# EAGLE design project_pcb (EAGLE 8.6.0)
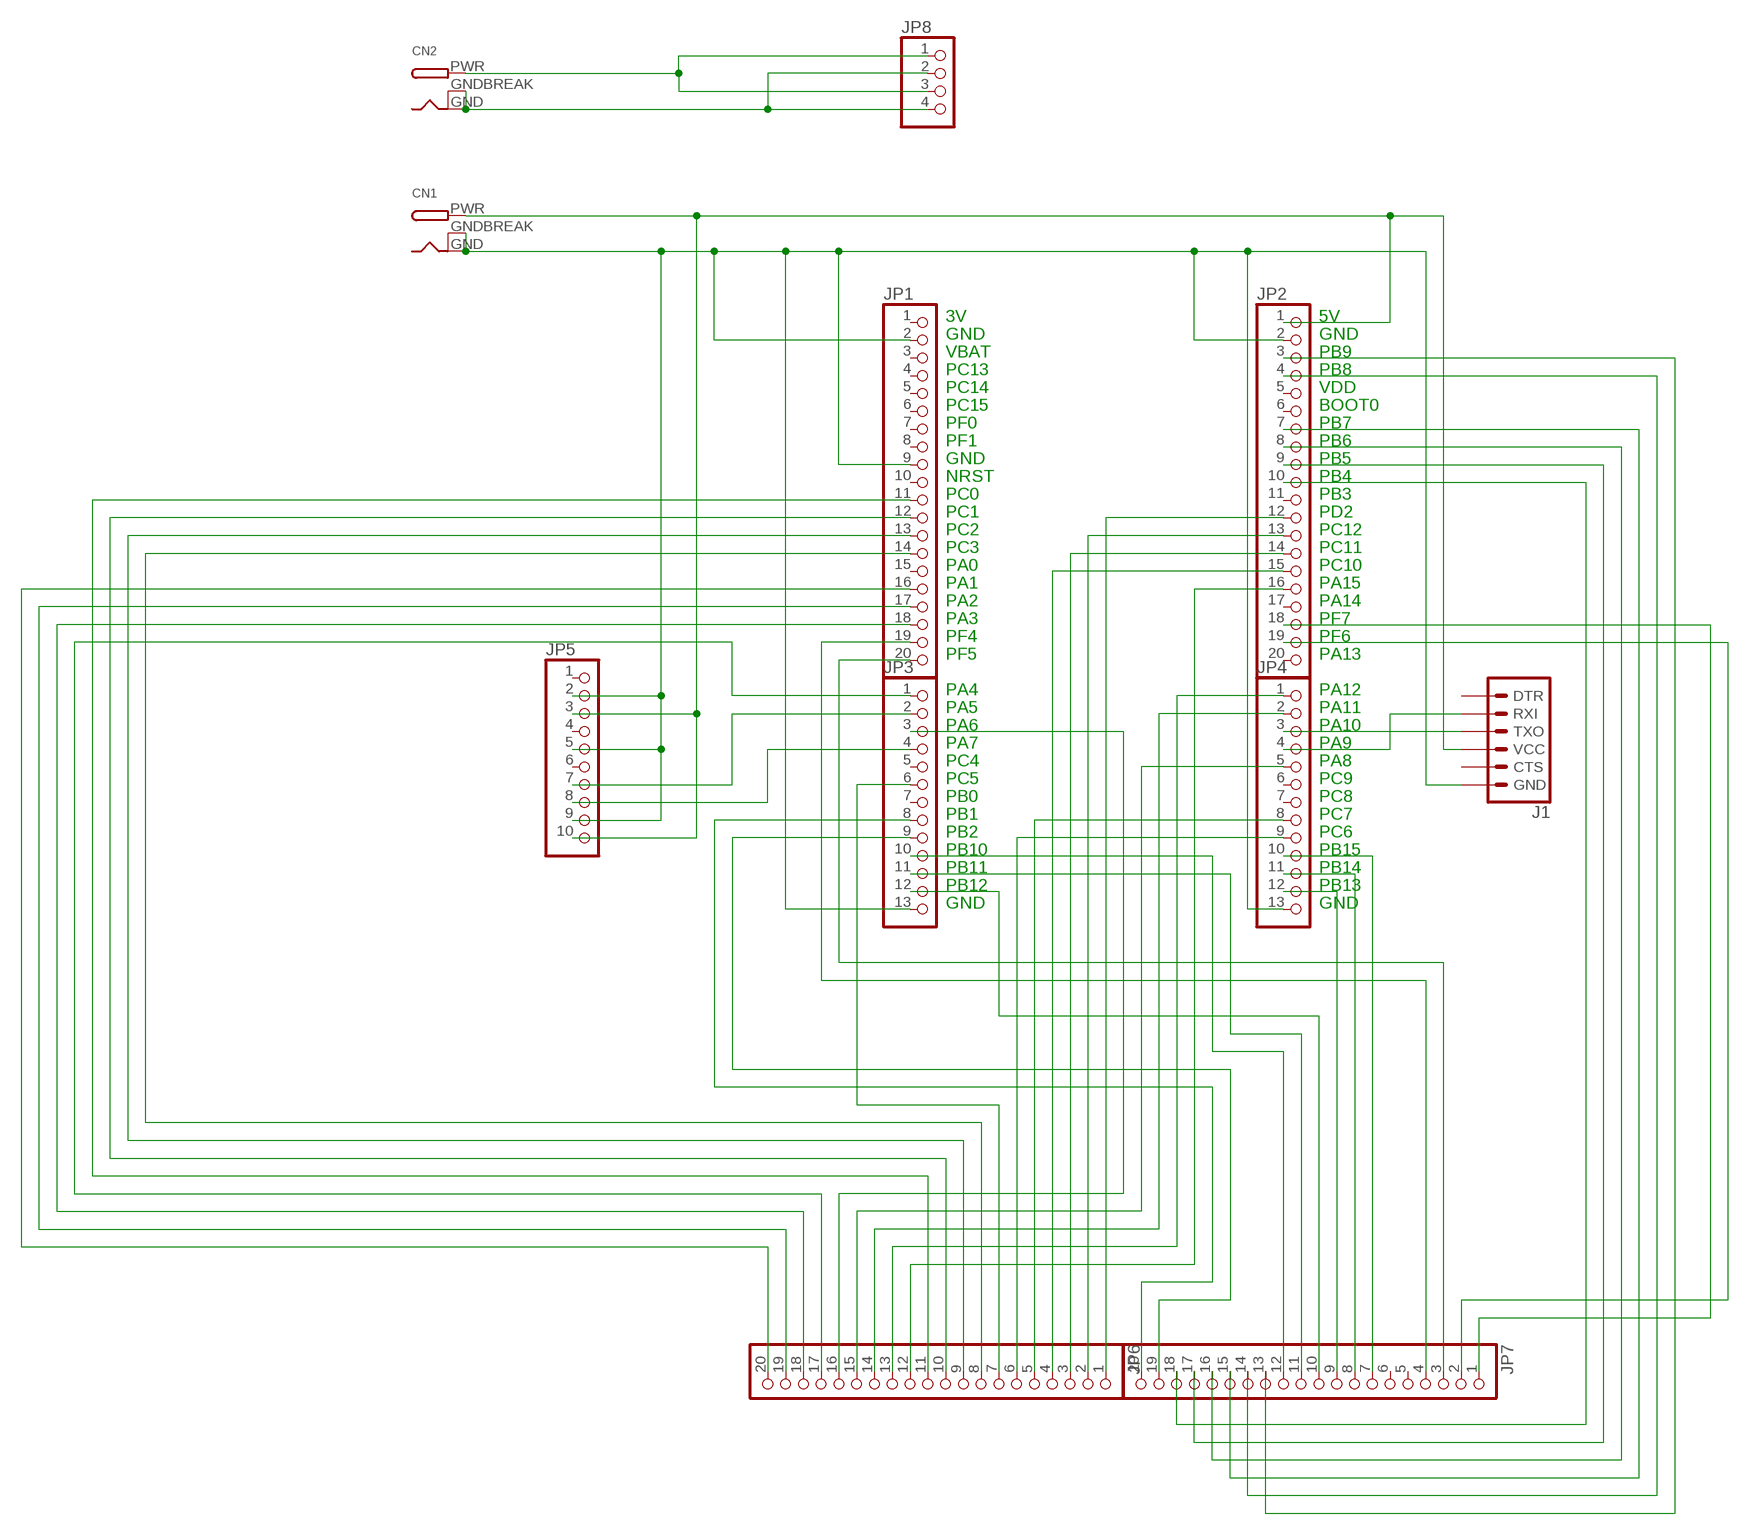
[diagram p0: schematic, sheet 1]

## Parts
CN1  DCBARRELPTH  [DCJACK_2MM_PTH]
CN2  DCBARRELPTH  [DCJACK_2MM_PTH]
J1  6_PIN_SERIAL_TARGET  [1X06]
JP1  PINHD-1X20  [1X20]
JP2  PINHD-1X20  [1X20]
JP3  PINHD-1X13  [1X13]
JP4  PINHD-1X13  [1X13]
JP5  PINHD-1X10  [1X10]
JP6  PINHD-1X20  [1X20]
JP7  PINHD-1X20  [1X20]
JP8  PINHD-1X4  [1X04]

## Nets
N$1: J1.3(TXO) JP4.3
N$2: J1.2(RXI) JP4.4
N$3: CN1.PWR J1.4(VCC) JP2.1 JP5.3 JP5.10
N$4: CN1.GND CN1.GNDBREAK J1.6(GND) JP1.2 JP1.9 JP2.2 JP3.13 JP4.13 JP5.2 JP5.5 JP5.9
N$5: JP3.2 JP5.7
N$6: JP3.4 JP5.8
N$7: JP1.16 JP6.20
N$8: JP1.17 JP6.19
N$9: JP1.18 JP6.18
N$10: JP3.1 JP6.17
N$11: JP3.3 JP6.16
N$12: JP4.5 JP6.15
N$13: JP4.2 JP6.14
N$14: JP4.1 JP6.13
N$15: JP2.16 JP6.12
N$16: JP1.11 JP6.11
N$17: JP1.12 JP6.10
N$18: JP1.13 JP6.9
N$19: JP1.14 JP6.8
N$20: JP3.6 JP6.7
N$21: JP4.9 JP6.6
N$22: JP4.8 JP6.5
N$23: JP2.15 JP6.4
N$24: JP2.14 JP6.3
N$25: JP2.13 JP6.2
N$26: JP2.10 JP7.18
N$27: JP3.8 JP7.20
N$28: JP3.9 JP7.19
N$29: JP2.9 JP7.17
N$30: JP2.8 JP7.16
N$31: JP2.7 JP7.15
N$32: JP2.4 JP7.14
N$33: JP2.3 JP7.13
N$34: JP3.10 JP7.12
N$35: JP3.11 JP7.11
N$36: JP3.12 JP7.10
N$37: JP4.12 JP7.9
N$38: JP4.11 JP7.8
N$39: JP4.10 JP7.7
N$40: JP2.18 JP7.1
N$41: JP2.19 JP7.2
N$42: JP1.20 JP7.3
N$43: JP1.19 JP7.4
N$44: JP2.12 JP6.1
N$45: CN2.GND CN2.GNDBREAK JP8.2 JP8.4
N$46: CN2.PWR JP8.1 JP8.3
Unconnected: J1.1(DTR) J1.5(CTS) JP1.1 JP1.3 JP1.4 JP1.5 JP1.6 JP1.7 JP1.8 JP1.10 JP1.15 JP2.5 JP2.6 JP2.11 JP2.17 JP2.20 JP3.5 JP3.7 JP4.6 JP4.7 JP5.1 JP5.4 JP5.6 JP7.5 JP7.6

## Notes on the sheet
- 3V | 5V
- GND | GND
- VBAT | PB9
- PC13 | PB8
- PC14 | VDD
- PC15 | BOOT0
- PF0 | PB7
- PF1 | PB6
- GND | PB5
- NRST | PB4
- PC0 | PB3
- PC1 | PD2
- PC2 | PC12
- PC3 | PC11
- PA0 | PC10
- PA1 | PA15
- PA2 | PA14
- PA3 | PF7
- PF4 | PF6
- PF5 | PA13
- PA4 | PA12
- PA5 | PA11
- PA6 | PA10
- PA7 | PA9
- PC4 | PA8
- PC5 | PC9
- PB0 | PC8
- PB1 | PC7
- PB2 | PC6
- PB10 | PB15
- PB11 | PB14
- PB12 | PB13
- GND | GND

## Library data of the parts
CN1 CN2 = adafruit:DCBARREL: 2.0mm DC Barrel Jack DCJACK_2MM_PTH - Through Hole Jack (4UConnector: 05537)
J1 = SparkFun-Connectors:6_PIN_SERIAL_TARGET: 6-pin header connection for use with the "FTDI BASIC" pinout - TARGET SIDE. Also known as "Arduino Serial Program Header". It is used to mate with our FTDI Basic serial programmers using the Arduino IDE. Note, this device has "TARGET" in the name. It is intended to be used on a design that contains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
JP1 JP2 JP6 JP7 = pinhead:PINHD-1X20: PIN HEADER
JP3 JP4 = pinhead:PINHD-1X13: PIN HEADER
JP5 = pinhead:PINHD-1X10: PIN HEADER
JP8 = pinhead:PINHD-1X4: PIN HEADER

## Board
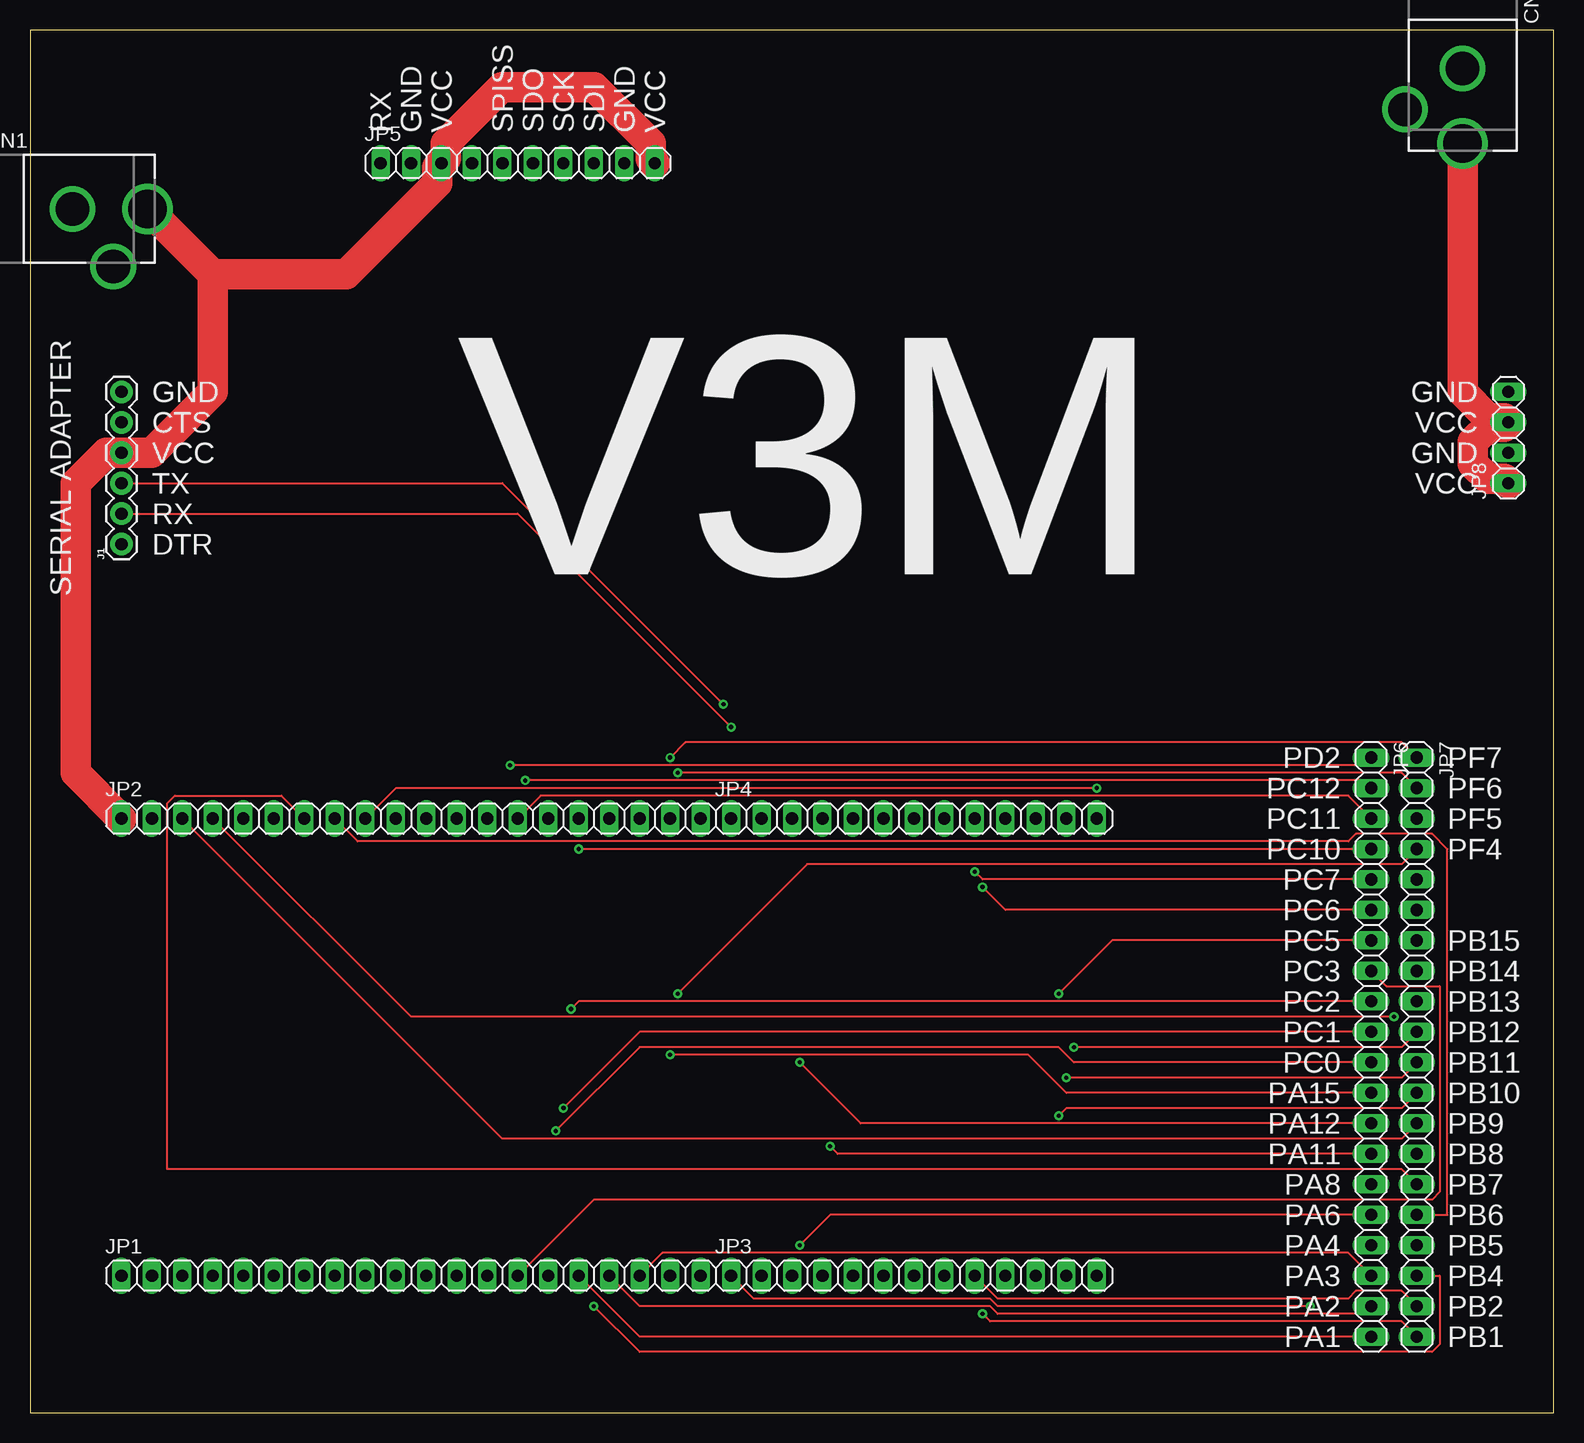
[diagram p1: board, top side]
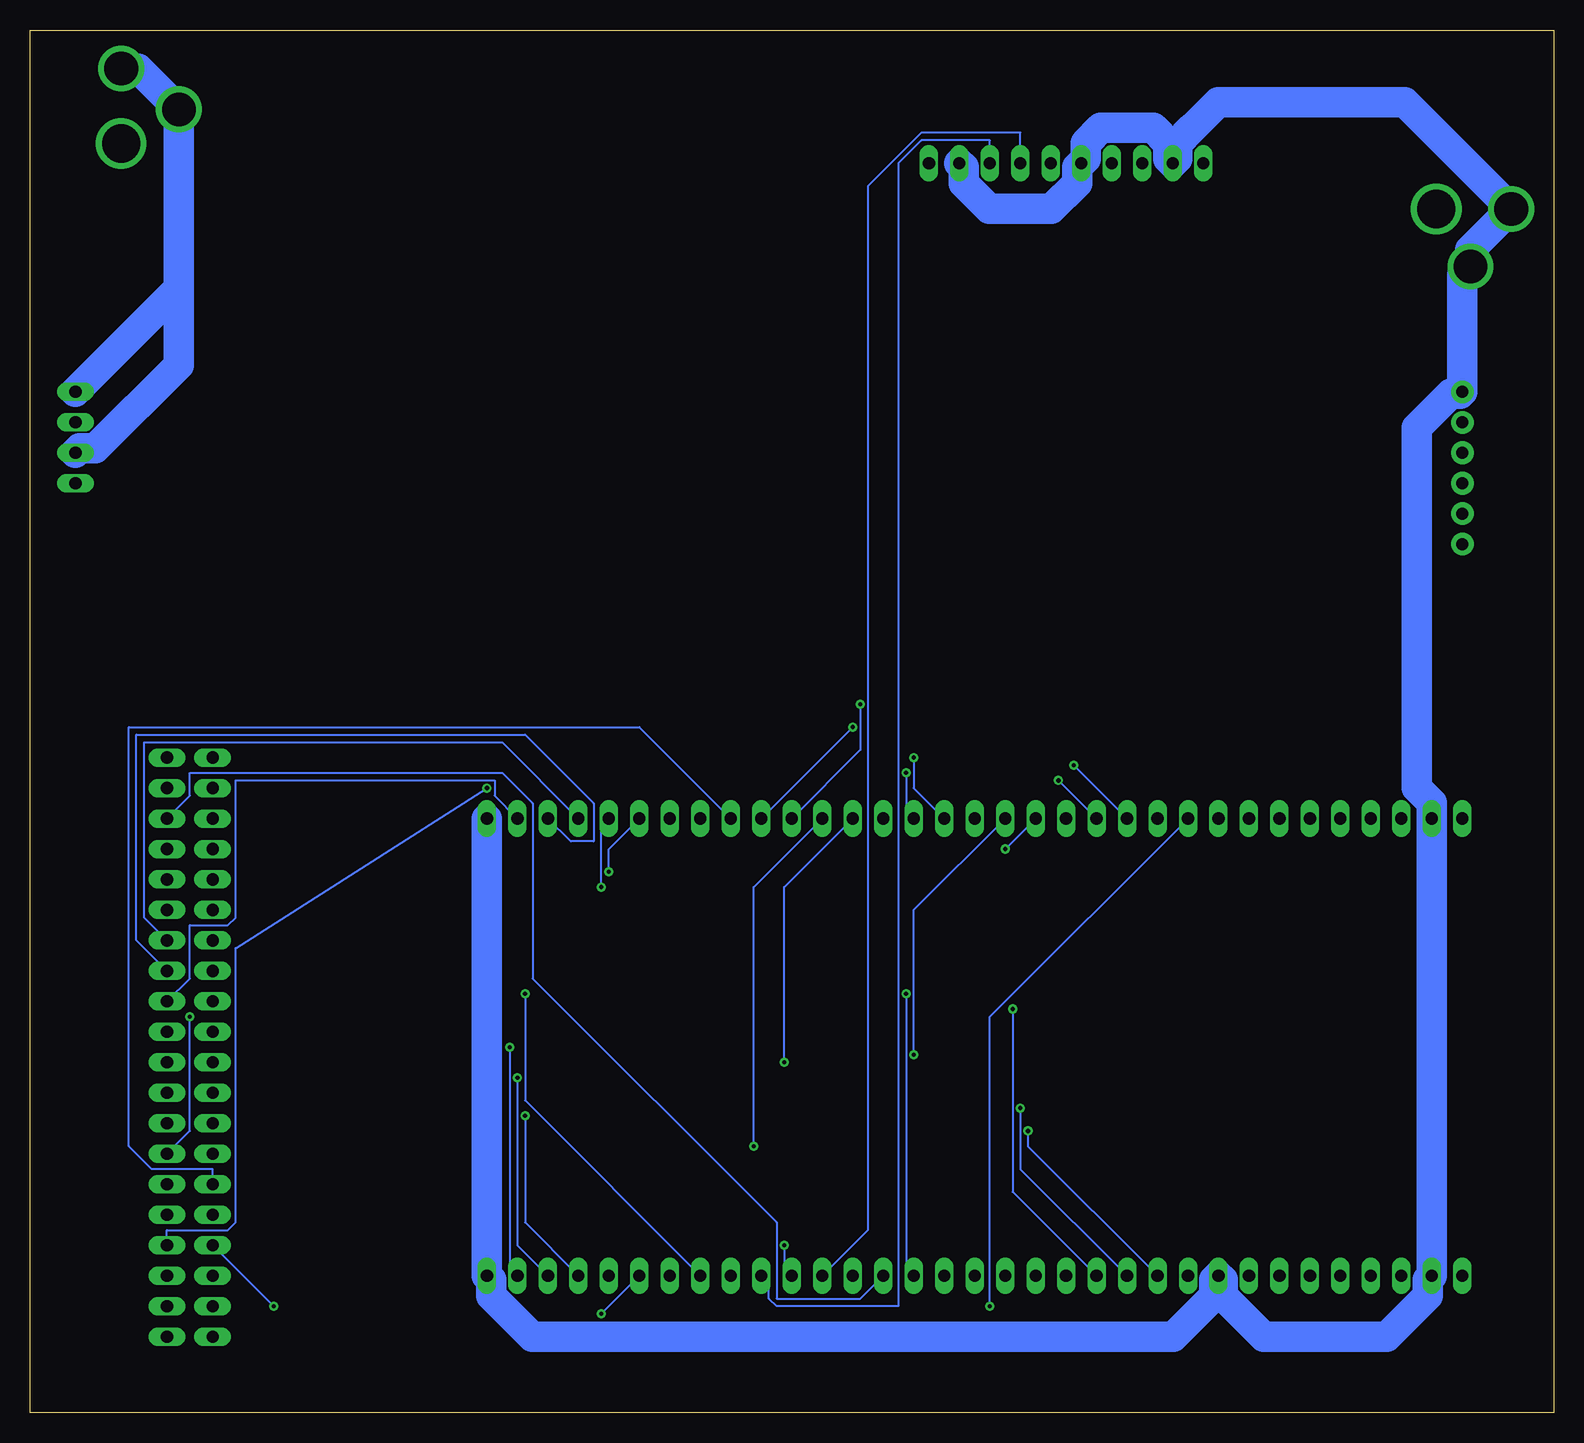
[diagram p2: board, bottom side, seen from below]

Size 126.98 x 115.24 mm. Coordinates in mm from the lower left corner, seen from the top.
Outline: 0,0 126.98,0 126.98,115.24 0,115.24 0,0
Copper layers (1*16): Top 0.035mm / dielectric 1.5mm / Bottom 0.035mm
Design rules "default": minimum track width 6mil, minimum drill 0.35mm, track to track 6mil, track to pad 6mil, pad to pad 6mil, via to via 6mil, smd to smd 6mil, copper to edge 40mil, drill to drill 6mil, minimum pad ring 10mil, minimum via ring 8mil, stop-mask expansion 4mil, vias tented up to drill 0mil, thermal gap 10mil

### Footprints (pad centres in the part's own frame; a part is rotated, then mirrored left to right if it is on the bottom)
DCJACK_2MM_PTH = drill 2.8: GND 0,7.35; GNDBREAK 4.8,10.75 | drill 3.2: PWR 0,13.6
1X06 = drill 1.016 pad 1.88: 1 0,0; 2 2.54,0; 3 5.08,0; 4 7.62,0; 5 10.16,0; 6 12.7,0
1X20 = drill 1.016 long: 1 -24.13,0; 2 -21.59,0; 3 -19.05,0; 4 -16.51,0; 5 -13.97,0; 6 -11.43,0; 7 -8.89,0; 8 -6.35,0; 9 -3.81,0; 10 -1.27,0; 11 1.27,0; 12 3.81,0; 13 6.35,0; 14 8.89,0; 15 11.43,0; 16 13.97,0; 17 16.51,0; 18 19.05,0; 19 21.59,0; 20 24.13,0
1X13 = drill 1.016 long: 1 -15.24,0; 2 -12.7,0; 3 -10.16,0; 4 -7.62,0; 5 -5.08,0; 6 -2.54,0; 7 0,0; 8 2.54,0; 9 5.08,0; 10 7.62,0; 11 10.16,0; 12 12.7,0; 13 15.24,0
1X10 = drill 1.016 long: 1 -11.43,0; 2 -8.89,0; 3 -6.35,0; 4 -3.81,0; 5 -1.27,0; 6 1.27,0; 7 3.81,0; 8 6.35,0; 9 8.89,0; 10 11.43,0
1X04 = drill 1.016 long: 1 -3.81,0; 2 -1.27,0; 3 1.27,0; 4 3.81,0

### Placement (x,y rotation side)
CN1  -3.81,100.33 270 top
CN2  119.38,119.38 180 top
J1  7.62,72.39 90 top
JP1  31.75,11.43 0 top
JP2  31.75,49.53 0 top
JP3  73.66,11.43 0 top
JP4  73.66,49.53 0 top
JP5  40.64,104.14 0 top
JP6  111.76,30.48 270 top
JP7  115.57,30.48 270 top
JP8  123.19,81.28 90 top

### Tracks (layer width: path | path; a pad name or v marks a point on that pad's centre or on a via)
N$1  (via drill 0.35)
  Top 0.152: v57.78,59.05 39.37,77.47 J1.3
  Bottom 0.152: JP4.3 57.78,55.24 v57.78,59.05
N$2  (via drill 0.35)
  Top 0.152: v58.42,57.15 40.64,74.93 J1.2
  Bottom 0.152: v58.42,57.15 JP4.4
N$3
  Top 2.54: CN1.PWR 15.24,94.88 | 15.24,94.88 15.24,85.09 10.16,80.01 J1.4 6.35,80.01 3.81,77.47 3.81,53.34 JP2.1 | 15.24,94.88 26.34,94.88 33.93,102.47 33.93,103.78 JP5.3 34.65,104.5 34.65,105.81 39.33,110.49 47.03,110.49 51.71,105.81 51.71,104.5 JP5.10
N$4
  Bottom 2.54: JP4.13 JP3.13 88.54,11.07 88.54,9.76 85.13,6.35 31.71,6.35 28.3,9.76 28.3,11.07 JP1.9 27.58,11.07 27.58,9.76 24.17,6.35 13.93,6.35 10.52,9.76 10.52,11.07 JP1.2 JP2.2 10.16,50.84 11.41,52.09 11.41,82.1 8.6,84.91 7.8,84.91 J1.6 7.62,94.85 CN1.GNDBREAK 6.94,96.93 CN1.GND 12.43,109.22 27.94,109.22 30.07,107.09 30.11,107.09 31.39,105.81 31.39,104.5 JP5.2 32.11,104.5 32.11,105.81 33.38,107.09 37.73,107.09 39.01,105.81 39.01,104.5 JP5.5 39.73,103.78 39.73,102.47 41.87,100.33 47.03,100.33 49.17,102.47 49.17,103.78 JP5.9
N$5
  Bottom 0.152: JP3.2 57.15,15.24 57.15,102.23 52.7,106.68 44.45,106.68 JP5.7
N$6
  Bottom 0.152: JP3.4 65.41,10.79 65.41,9.53 64.77,8.89 54.61,8.89 54.61,104.14 52.7,106.05 46.99,106.05 JP5.8
N$7
  Top 0.152: JP1.16 50.8,6.35 JP6.20
N$8
  Top 0.152: JP1.17 50.8,8.89 80.01,8.89 80.64,8.26 111.12,8.26 JP6.19
N$9
  Top 0.152: JP1.18 52.7,13.34 109.86,13.34 JP6.18
N$10  (via drill 0.35)
  Top 0.152: JP3.1 60.33,9.53 80.01,9.53 80.64,8.89 v106.68,8.89
  Bottom 0.152: JP6.17 v106.68,8.89
N$11  (via drill 0.35)
  Top 0.152: v64.14,13.97 66.67,16.51 JP6.16
  Bottom 0.152: JP3.3 64.14,12.06 v64.14,13.97
N$12
  Bottom 0.152: JP4.5 76.2,57.15 118.75,57.15 118.75,22.23 116.84,20.32 111.76,20.32 JP6.15
N$13  (via drill 0.35)
  Top 0.152: v66.67,22.23 67.31,21.59 JP6.14
  Bottom 0.152: JP4.2 66.67,43.81 v66.67,22.23
N$14  (via drill 0.35)
  Top 0.152: v64.14,29.21 69.22,24.13 JP6.13
  Bottom 0.152: JP4.1 64.14,43.81 v64.14,29.21
N$15  (via drill 0.35)
  Top 0.152: v53.34,29.84 83.19,29.84 86.36,26.67 JP6.12
  Bottom 0.152: JP2.16 53.34,41.91 v53.34,29.84
N$16  (via drill 0.35)
  Top 0.152: v43.81,23.5 50.8,30.48 85.72,30.48 87,29.21 JP6.11
  Bottom 0.152: JP1.11 43.81,22.23 v43.81,23.5
N$17  (via drill 0.35)
  Top 0.152: v44.45,25.4 50.8,31.75 JP6.10
  Bottom 0.152: JP1.12 44.45,20.32 v44.45,25.4
N$18  (via drill 0.35)
  Top 0.152: v45.09,33.66 45.72,34.29 JP6.9
  Bottom 0.152: JP1.13 45.09,18.41 v45.09,33.66
N$19
  Top 0.152: JP1.14 46.99,17.78 116.84,17.78 117.47,18.41 117.47,35.56 113.03,35.56 JP6.8
N$20  (via drill 0.35)
  Top 0.152: v85.72,34.92 90.17,39.37 JP6.7
  Bottom 0.152: JP3.6 85.72,26.04 v85.72,34.92
N$21  (via drill 0.35)
  Top 0.152: v79.38,43.81 81.28,41.91 JP6.6
  Bottom 0.152: JP4.9 79.38,48.9 v79.38,43.81
N$22  (via drill 0.35)
  Top 0.152: v78.74,45.09 79.38,44.45 JP6.5
  Bottom 0.152: JP4.8 78.74,46.99 v78.74,45.09
N$23  (via drill 0.35)
  Top 0.152: JP6.4 v45.72,46.99
  Bottom 0.152: v45.72,46.99 JP2.15
N$24
  Top 0.152: JP2.14 42.55,51.44 109.86,51.44 JP6.3
N$25  (via drill 0.35)
  Top 0.152: v41.27,52.7 111.12,52.7 JP6.2
  Bottom 0.152: v41.27,52.7 JP2.13
N$26  (via drill 0.35)
  Top 0.152: v46.99,8.89 50.8,5.08 116.84,5.08 117.47,5.71 117.47,11.43 JP7.18
  Bottom 0.152: JP2.10 46.99,33.02 v46.99,8.89
N$27  (via drill 0.35)
  Top 0.152: v79.38,8.26 80.01,7.62 114.3,7.62 JP7.20
  Bottom 0.152: v79.38,8.26 JP3.8
N$28
  Top 0.152: JP3.9 80.64,9.53 109.86,9.53 110.49,10.16 114.3,10.16 JP7.19
N$29  (via drill 0.35)
  Top 0.152: JP2.9 30.48,52.07 v88.9,52.07
  Bottom 0.152: v88.9,52.07 109.86,38.73 109.86,15.88 110.49,15.24 115.57,15.24 JP7.17
N$30
  Top 0.152: JP2.8 27.3,47.62 109.86,47.62 110.49,48.26 116.84,48.26 118.11,46.99 118.11,16.51 JP7.16
N$31
  Top 0.152: JP2.7 20.95,51.44 12.06,51.44 11.43,50.8 11.43,20.32 114.3,20.32 JP7.15
N$32  (via drill 0.35)
  Top 0.152: JP2.4 31.75,33.02 v113.67,33.02
  Bottom 0.152: v113.67,33.02 113.67,23.5 JP7.14
N$33
  Top 0.152: JP2.3 39.37,22.86 114.3,22.86 JP7.13
N$34  (via drill 0.35)
  Top 0.152: v85.72,24.77 86.36,25.4 114.3,25.4 JP7.12
  Bottom 0.152: JP3.10 85.72,15.88 v85.72,24.77
N$35  (via drill 0.35)
  Top 0.152: v86.36,27.94 114.3,27.94 JP7.11
  Bottom 0.152: JP3.11 86.36,13.97 v86.36,27.94
N$36  (via drill 0.35)
  Top 0.152: v87,30.48 114.3,30.48 JP7.10
  Bottom 0.152: JP3.12 87,12.06 v87,30.48
N$37
  Bottom 0.152: JP4.12 88.27,51.44 88.27,52.7 109.86,52.7 109.86,41.27 110.49,40.64 113.67,40.64 113.67,36.2 JP7.9
N$38
  Bottom 0.152: JP4.11 81.92,47.62 80.01,47.62 80.01,50.8 85.72,56.52 118.11,56.52 118.11,39.37 JP7.8
N$39
  Bottom 0.152: JP4.10 87.63,55.88 117.47,55.88 117.47,41.27 JP7.7
N$40  (via drill 0.35)
  Top 0.152: v53.34,54.61 54.61,55.88 114.3,55.88 JP7.1
  Bottom 0.152: JP2.18 53.34,52.07 v53.34,54.61
N$41  (via drill 0.35)
  Top 0.152: v53.98,53.34 114.3,53.34 JP7.2
  Bottom 0.152: JP2.19 53.98,50.16 v53.98,53.34
N$42
  Bottom 0.152: JP1.20 57.78,9.53 64.77,9.53 64.77,15.88 85.09,36.2 85.09,50.8 87.63,53.34 113.67,53.34 113.67,51.44 JP7.3
N$43  (via drill 0.35)
  Top 0.152: v53.98,34.92 64.77,45.72 114.3,45.72 JP7.4
  Bottom 0.152: JP1.19 53.98,12.06 v53.98,34.92
N$44  (via drill 0.35)
  Top 0.152: v40.01,53.98 111.12,53.98 JP6.1
  Bottom 0.152: v40.01,53.98 JP2.12
N$45
  Bottom 2.54: CN2.GND 117.98,112.03 CN2.GNDBREAK 114.58,93.7 | 114.58,93.7 JP8.4 | JP8.2 122.83,80.37 121.52,80.37 114.58,87.31 114.58,93.7
N$46
  Top 2.54: CN2.PWR 119.38,85.05 121.52,82.91 122.83,82.91 JP8.3 122.83,82.19 121.52,82.19 120.24,80.92 120.24,79.11 121.52,77.83 122.83,77.83 JP8.1

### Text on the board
tPlace: RX | GND | VCC | SPISS | SDO | SCK | SDI | GND | VCC | GND | GND | CTS | VCC | VCC | GND | SERIAL ADAPTER | TX | VCC | RX | DTR | V3M | PD2 | PF7 | PC12 | PF6 | PC11 | PF5 | PC10 | PF4 | PC7 | PC6 | PC5 | PB15 | PC3 | PB14 | PC2 | PB13 | PC1 | PB12 | PC0 | PB11 | PA15 | PB10 | PA12 | PB9 | PA11 | PB8 | PA8 | PB7 | PA6 | PB6 | PA4 | PB5 | PA3 | PB4 | PA2 | PB2 | PA1 | PB1

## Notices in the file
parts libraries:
SparkFun-Connectors: Licensing: Creative Commons ShareAlike 4.0 International - https://creativecommons.org/licenses/by-sa/4.0
